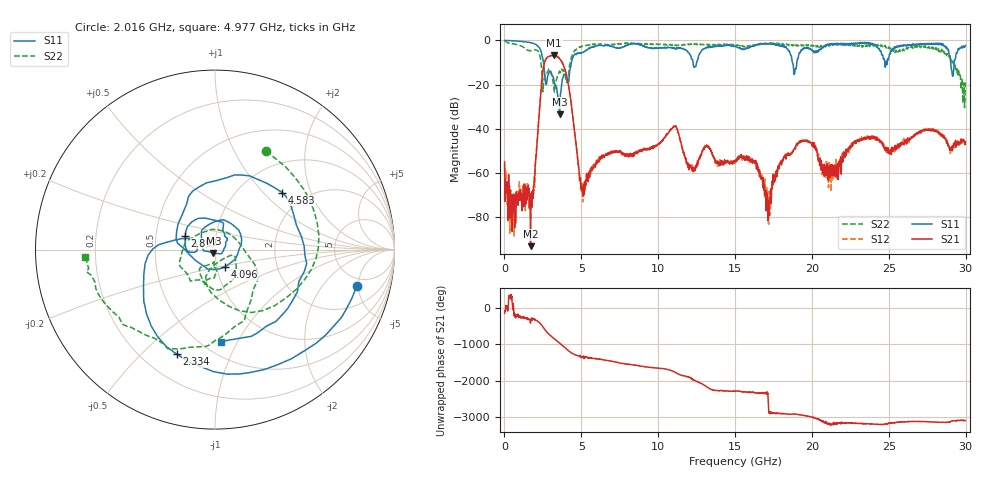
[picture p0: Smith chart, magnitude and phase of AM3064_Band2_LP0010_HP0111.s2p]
# Hz S DB R 50.0
!freq dBS11 angS11 dBS21 angS21 dBS12 angS12 dBS22 angS22
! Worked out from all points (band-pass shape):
!   1600 points, 10 MHz to 29.98 GHz, reference 50 ohm
!   highest |S21| = -6.71 dB at 3.234 GHz (marker M1); lowest = -93.2 dB at 1.697 GHz (marker M2)
!   |S21| within 3 dB of the highest: 2.622 GHz to 3.727 GHz (1.105 GHz wide, 34.8 % of centre)
!   lowest |S11| = -33.4 dB at 3.59 GHz (marker M3), VSWR 1.04, Z = 49.1 - j1.91 ohm
!   |S11| at or under -10 dB: 2.539 GHz to 4.35 GHz (1.811 GHz wide, 52.6 % of centre); 12.26 GHz to 12.5 GHz (240.1 MHz wide, 1.94 % of centre); 18.73 GHz to 19.02 GHz (291.7 MHz wide, 1.55 % of centre)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
!   |S22| runs from -30.4 to -0.2 dB; largest |S21 - S12| = 0.0098
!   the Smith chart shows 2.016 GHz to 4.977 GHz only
!   S11 on the Smith chart (normalised r, x): 2.016 GHz: 3.87, -4.74; 2.334 GHz: 0.34, -0.64; 2.897 GHz: 0.71, +0.12; 4.096 GHz: 1.09, -0.21; 4.583 GHz: 1.54, +1.29; 4.977 GHz: 0.62, -0.86
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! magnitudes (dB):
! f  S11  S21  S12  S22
! 10 MHz  0.0  -55.0  -56.2  -0.2
! 591.1 MHz  -0.2  -69.7  -78.9  -1.6
! 1.697 GHz  -1.1  -93.2  -70.8  -4.6
! 2.016 GHz  -1.8  -55.8  -55.5  -4.2
! 2.334 GHz  -4.1  -26.1  -26.1  -7.9
! 2.897 GHz  -14.7  -7.3  -7.2  -12.9
! 3.234 GHz  -18.6  -6.7  -6.8  -22.8
! 3.59 GHz  -33.4  -8.3  -8.4  -13.9
! 4.096 GHz  -19.1  -17.8  -17.6  -18.6
! 4.583 GHz  -6.2  -42.6  -42.7  -4.4
! 4.977 GHz  -5.8  -67.2  -65.3  -2.8
! 5.015 GHz  -5.8  -66.6  -67.7  -2.9
! 10 GHz  -3.5  -47.0  -47.2  -1.8
! 15 GHz  -2.5  -54.6  -55.0  -1.9
! 16.3 GHz  -2.1  -54.5  -55.4  -2.1
! 17.14 GHz  -1.6  -81.7  -74.5  -1.3
! 19.99 GHz  -4.1  -46.6  -47.0  -2.1
! 21.28 GHz  -1.7  -57.9  -63.5  -1.7
! 23.16 GHz  -1.1  -45.1  -45.0  -2.9
! 25 GHz  -8.0  -51.1  -51.0  -3.0
! 28.56 GHz  -2.2  -43.8  -42.9  -4.8
! 29.98 GHz  -2.3  -46.0  -47.4  -19.1
